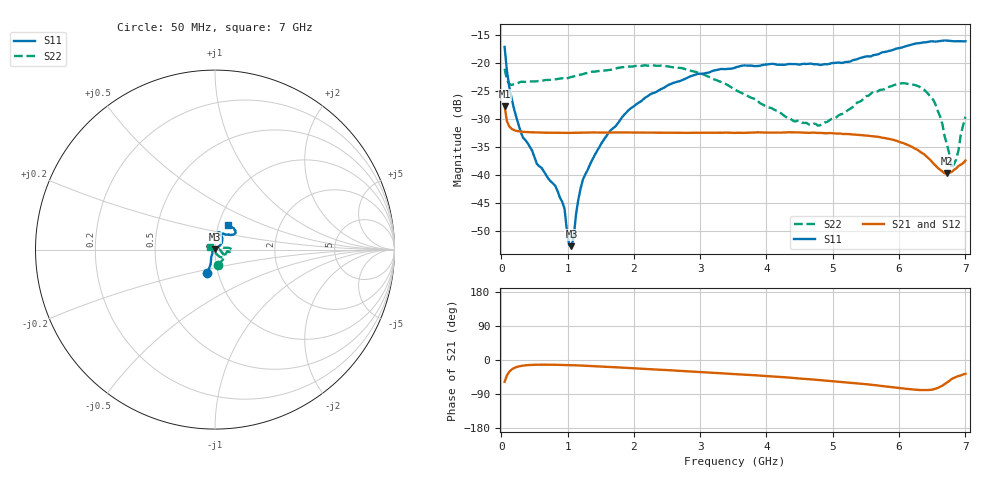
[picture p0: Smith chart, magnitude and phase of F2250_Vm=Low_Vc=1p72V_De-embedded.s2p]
! Integrated Device Technology
! Corporate Headquarters
! 6024 Silver Creek Valley Road
! San Jose, CA 95138  USA
! Phone:  1-408-284-8200
! Toll Free:  1-800-223-1366
! Webpage:  http://www.idt.com/
! Timing and RF Division
! 515 Groton Road, Suite 102
! Westford, MA 01886-6024
! Device:  F2250
! Description: Voltage Variable RF Attenuator
! Frequency:  50.0 -  6000.00 MHz
! Package:  3x3 mm Thin QFN Plastic Package: 16 pin
! Ports:  2 RF, 3 DC
!  Pin  1  = GND
!  Pin  2  = NC
!  Pin  3  = RF1  = Port 1
!  Pin  4  = NC
!  Pin  5  = GND
!  Pin  6  = GND
!  Pin  7  = GND
!  Pin  8  = GND
!  Pin  9  = NC
!  Pin 10  = RF2  = Port 2
!  Pin 11  = NC
!  Pin 12  = GND
!  Pin 13  = GND
!  Pin 14  = VCNTRL
!  Pin 15  = VDD
!  Pin 16  = VMODE
! Vcntrl:  1.720 Volts
! Vmode:  +0.000 Volts
! Vdd:  +3.30  Volts
! Current:  1.187 mA
! Data:  The device was measured on a the F2250 evaluation board which has
!  individual transmission lines to the RF pins.  Data was collected
!  using a calibrated network analyzer.  The evaluation board was
!  de-embedded using a TRL calibration technique.
!  The reference plane is the edge of the package pin.
! Misc:  SN 10
!  Action Tracker AT0258
! Date Measured:  2014-11-26
! Date:  2015-10-15  MJV
! Note:
!  Integrated Device Technology supplies this data as a sample of measured
!  data at the package pin for this product.  Your particular data for this
!  product may vary.
!  Data was taken at 25 degrees C.
!  Integrated Device Technology reserves the right to change this data at anytime.
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# GHz S dB R 50
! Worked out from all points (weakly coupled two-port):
!   201 points, 50 MHz to 7 GHz, reference 50 ohm
!   highest |S21| = -27.71 dB at 50 MHz (marker M1); lowest = -39.7 dB at 6.722 GHz (marker M2)
!   lowest |S11| = -52.6 dB at 1.058 GHz (marker M3), VSWR 1.00, Z = 49.9 + j0.217 ohm
!   |S11| at or under -10 dB: start of sweep to end of sweep
!   |S22| runs from -38.8 to -20.4 dB; largest |S21 - S12| = 8.9e-05
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0.05  -17.16 -108.1  -27.71 -57.6  -27.71 -57.6  -21.04 -79.8
0.1195  -24.20 -110.9  -31.31 -31.1  -31.31 -31.0  -23.74 -31.4
0.29325  -32.31 -125.9  -32.24 -15.8  -32.23 -15.8  -23.38 -13.7
0.5365  -37.98 -153.3  -32.39 -12.4  -32.37 -12.5  -23.28 -7.9
0.8145  -41.90 173.6  -32.44 -12.6  -32.44 -12.6  -22.93 -8.7
0.9535  -45.96 171.4  -32.46 -13.2  -32.46 -13.2  -22.91 -9.3
1.023  -52.44 139.3  -32.47 -13.5  -32.46 -13.5  -22.62 -8.7
1.05775  -52.64 111.3  -32.46 -13.7  -32.45 -13.7  -22.52 -8.6
1.0925  -50.96 74.0  -32.45 -13.9  -32.44 -13.9  -22.41 -8.9
1.162  -44.30 49.2  -32.44 -14.3  -32.44 -14.3  -22.18 -9.6
1.2315  -40.79 39.4  -32.41 -14.8  -32.44 -14.8  -22.01 -10.0
1.6485  -32.02 40.2  -32.40 -18.4  -32.41 -18.4  -21.24 -7.5
2.37825  -24.87 46.6  -32.43 -25.5  -32.45 -25.5  -20.51 -2.0
3.525  -20.85 72.1  -32.47 -37.1  -32.47 -37.1  -24.78 9.7
4.7065  -20.23 72.1  -32.42 -51.5  -32.43 -51.5  -30.84 5.2
5.85325  -17.85 40.2  -33.56 -70.9  -33.57 -70.9  -24.25 -35.8
6.40925  -16.33 41.6  -36.62 -79.4  -36.65 -79.3  -25.14 -50.9
6.54825  -16.21 44.9  -38.26 -75.7  -38.28 -75.7  -27.39 -59.0
6.722  -16.03 50.0  -39.68 -59.1  -39.67 -59.0  -34.53 -85.6
6.7915  -16.12 52.1  -39.45 -50.2  -39.47 -50.0  -38.84 -119.9
6.861  -16.15 54.9  -38.80 -44.6  -38.79 -44.5  -37.19 -161.5
7  -16.16 63.1  -37.39 -36.5  -37.34 -36.7  -29.60 155.8
